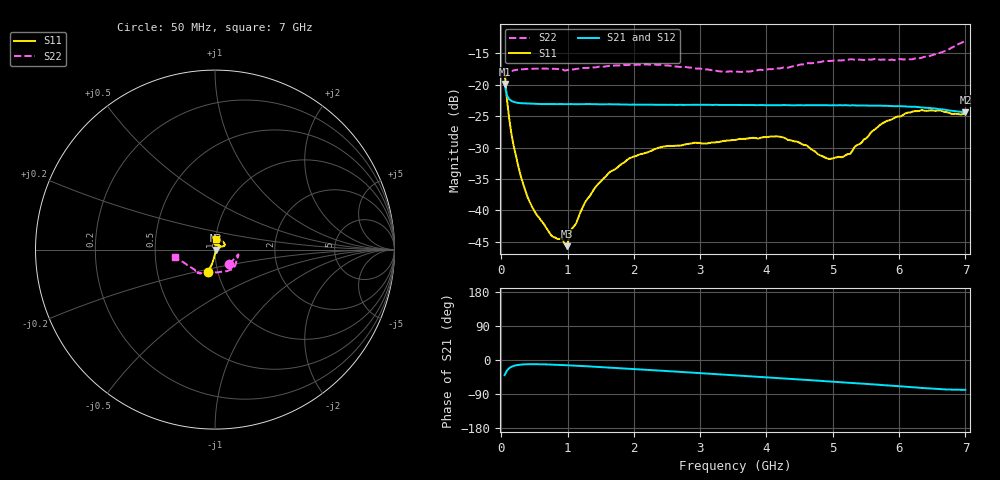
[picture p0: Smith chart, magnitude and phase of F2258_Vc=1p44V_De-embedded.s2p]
! Integrated Device Technology
! Corporate Headquarters
! 6024 Silver Creek Valley Road
! San Jose, CA 95138  USA
! Phone:  1-408-284-8200
! Toll Free:  1-800-223-1366
! Webpage:  http://www.idt.com/
! Timing and RF Division
! 515 Groton Road, Suite 102
! Westford, MA 01886-6024
! Device:  F2258
! Description: Voltage Variable RF Attenuator
! Frequency:  50.0 -  6000.00 MHz
! Package:  3x3 mm Thin QFN Plastic Package: 16 pin
! Ports:  2 RF, 2 DC
!  Pin  1  = NC
!  Pin  2  = NC
!  Pin  3  = RF2  = Port 2
!  Pin  4  = GND
!  Pin  5  = Vdd
!  Pin  6  = NC
!  Pin  7  = VCTRL
!  Pin  8  = NC
!  Pin  9  = GND
!  Pin 10  = RF1  = Port 1
!  Pin 11  = NC
!  Pin 12  = NC
!  Pin 13  = NC
!  Pin 14  = NC
!  Pin 15  = NC
!  Pin 16  = NC
! Vcntrl:  1.440 Volts
! Vdd:  +3.300 Volts
! Current:  1.159 mA
! Data:  The device was measured on a the F2258 evaluation board which has
!  individual transmission lines to the RF pins.  Data was collected
!  using a calibrated network analyzer.  The evaluation board was
!  de-embedded using a TRL calibration technique.
!  The reference plane is the edge of the package pin.
! Misc:  SN 10
!  Action Tracker AT0285
! Date Measured:  2014-12-10
! Date:  2016-01-13  MJV
! Note:
!  Integrated Device Technology supplies this data as a sample of measured
!  data at the package pin for this product.  Your particular data for this
!  product may vary.
!  Data was taken at 25 degrees C.
!  Integrated Device Technology reserves the right to change this data at anytime.
!Freq_(GHz)  S11M_(dB)  S11P_(deg)  S21M_(dB)  S21P_(deg)  S12M_(dB)  S12P_(deg)  S22M_(dB)  S22P_(deg)
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# GHz S dB R 50
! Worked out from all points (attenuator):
!   201 points, 50 MHz to 7 GHz, reference 50 ohm
!   highest |S21| = -19.89 dB at 50 MHz (marker M1); lowest = -24.4 dB at 7 GHz (marker M2)
!   lowest |S11| = -45.7 dB at 988.2 MHz (marker M3), VSWR 1.01, Z = 50.4 - j0.276 ohm
!   |S11| at or under -10 dB: start of sweep to end of sweep
!   |S22| runs from -19.1 to -12.9 dB; largest |S21 - S12| = 0.00027
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0.05  -17.76 -107.0  -19.89 -40.1  -19.87 -40.0  -19.05 -45.6
0.08475  -22.23 -101.2  -21.69 -28.0  -21.66 -28.0  -18.33 -23.6
0.15425  -27.91 -96.2  -22.58 -17.8  -22.56 -17.8  -17.80 -14.5
0.29325  -34.52 -88.0  -22.93 -12.2  -22.89 -12.2  -17.55 -11.9
0.3975  -37.91 -81.8  -22.98 -11.1  -22.96 -11.1  -17.47 -12.5
0.745  -43.89 -43.5  -23.05 -12.1  -23.07 -12.1  -17.45 -18.4
0.91875  -44.42 -8.9  -23.08 -13.3  -23.07 -13.3  -17.51 -22.6
0.98825  -45.71 -31.8  -23.07 -13.8  -23.07 -13.8  -17.68 -23.8
1.05775  -43.02 -15.9  -23.07 -14.4  -23.09 -14.4  -17.55 -25.0
1.2315  -39.42 0.9  -23.09 -16.0  -23.08 -16.0  -17.34 -28.4
1.44  -36.05 7.2  -23.10 -18.2  -23.08 -18.2  -17.19 -32.4
1.6485  -33.79 12.4  -23.10 -20.3  -23.11 -20.3  -16.98 -36.2
1.9265  -31.74 21.4  -23.16 -23.2  -23.14 -23.2  -16.83 -41.2
2.37825  -30.02 33.3  -23.19 -27.9  -23.18 -27.9  -16.81 -49.7
3.525  -28.79 84.2  -23.21 -40.5  -23.22 -40.5  -17.93 -84.3
4.1505  -28.20 102.4  -23.26 -47.5  -23.26 -47.5  -17.36 -106.9
4.7065  -30.46 92.1  -23.24 -53.8  -23.25 -53.8  -16.53 -118.7
4.94975  -31.82 72.8  -23.27 -56.6  -23.26 -56.6  -16.20 -121.4
5.15825  -31.46 52.6  -23.26 -59.1  -23.27 -59.1  -16.08 -123.1
5.85325  -25.65 22.5  -23.37 -67.5  -23.37 -67.4  -16.04 -129.8
6.33975  -24.02 29.8  -23.61 -73.7  -23.61 -73.8  -15.69 -142.1
7  -24.40 83.7  -24.37 -78.6  -24.37 -78.6  -12.93 -169.4
